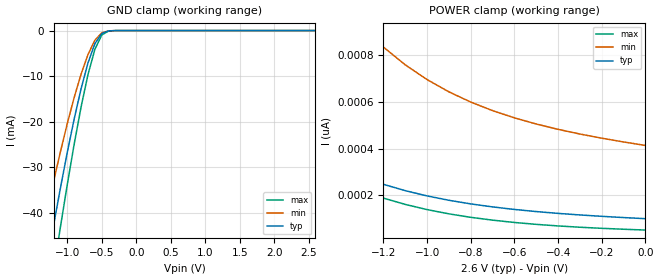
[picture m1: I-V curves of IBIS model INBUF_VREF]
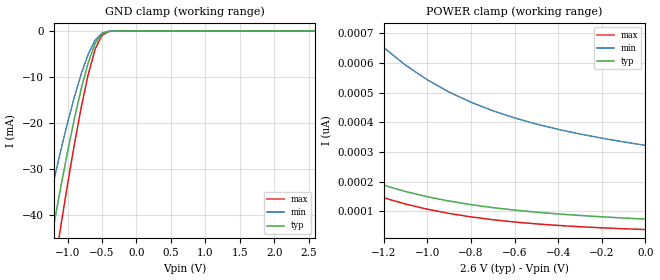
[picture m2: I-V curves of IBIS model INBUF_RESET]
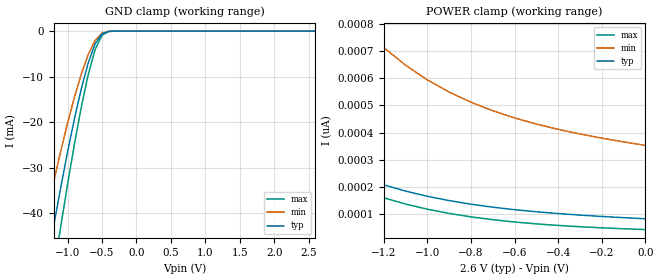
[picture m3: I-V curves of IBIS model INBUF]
| IBIS file sstvn859_tssop_3200.ibs created by s2ibis2 version 1.2
| North Carolina State University Electronics Research Laboratory  1995
[IBIS ver]   2.1
[File name]   sstvn859_tssop_3200.ibs
[File Rev]   1.0
[Date]   Thursday, November 6, 2003
[Source]   IDT
[Notes]   1. Temp typ=25C, min=0C, max=70C
   2. IDT's 2.0v C11.5 process
   3. Ramp rate based on 50 ohm load
READ THESE TERMS AND CONDITIONS CAREFULLY BEFORE USING THIS IBIS MODEL.  BY
USING THIS IBIS MODEL, YOU ARE ACCEPTING AND AGREEING TO THESE TERMS AND
CONDITIONS OF USE.
Integrated Device Technology, Inc. ("IDT") hereby grants the user of this
IBIS model ("User") a non-exclusive, nontransferable license to use this
IBIS model under the following terms: The User is granted this license only
to use the IBIS model for demonstration purposes only and is not granted
rights to sell, copy (except as needed to run the IBIS model), rent, lease
or sub-license (except for demonstration) the IBIS model in whole or in
part, or in modified form to anyone. The User may modify the IBIS model to
suit its specific applications, but  rights to derivative works and such
modifications shall belong to IDT.
THIS IBIS MODEL IS PROVIDED ON AN AS IS" BASIS AND IDT  MAKES ABSOLUTELY NO
WARRANTY WITH RESPECT TO THE INFORMATION CONTAINED HEREIN.  IDT DISCLAIMS
AND USER WAIVES ALL WARRANTIES, EXPRESS AND IMPLIED, INCLUDING WARRANTIES OF
MERCHANTABILITY AND FITNESS FOR A PARTICULAR PURPOSE.  THE ENTIRE RISK AS TO
QUALITY AND PERFORMANCE IS WITH THE USER  ACCORDINGLY, IN NO EVENT SHALL IDT
BE LIABLE FOR ANY DIRECT OR INDIRECT DAMAGES, WHETHER IN CONTRACT OR TORT,
INCLUDING ANY LOST PROFITS OR OTHER INCIDENTAL, CONSEQUENTIAL, EXEMPLARY, OR
PUNITIVE DAMAGES ARISING OUT OF THE USE OR APPLICATION OF THE  IBIS MODEL,
WHETHER OR NOT IDT HAD NOTICE OF SUCH DAMAGES.
IDT reserves the right to make changes without notice to any product herein
to improve reliability, function, or design. IDT does not convey any license
under patent rights or any other intellectual property rights, including
those of third parties. IDT is not obligated to provide maintenance or
support for the licensed IBIS model.
This model is for the 13-Bit to 26-Bit Registered Buffer With SSTL I/O
configuration
[Copyright]
Copyright 2002, Integrated Device Technology, Inc. All rights reserved.
|   Component IDT74SSTVN16859
[Component]   IDT74SSTVN16859
[Manufacturer]   Integrated Device Technology Inc.
[Package]
|Following package parameters are for TSSOP 64 lead package
| variable   typ   min   max
R_pkg   0.10500   68.00000m   0.14800
L_pkg   3.80000nH   2.05000nH   6.57000nH
C_pkg   0.22000pF   0.07183pF   0.42000pF
[Pin]  signal_name   model_name   R_pin   L_pin   C_pin
1   Q13A   OUTBUF
2   Q12A   OUTBUF
3   Q11A   OUTBUF
4   Q10A   OUTBUF
5   Q9A   OUTBUF
6   VDDQ   POWER
7   GND   GND
8   Q8A   OUTBUF
9   Q7A   OUTBUF
10   Q6A   OUTBUF
11   Q5A   OUTBUF
12   Q4A   OUTBUF
13   Q3A   OUTBUF
14   Q2A   OUTBUF
15   GND   GND
16   Q1A   OUTBUF
17   Q13B   OUTBUF
18   VDDQ   POWER
19   Q12B   OUTBUF
20   Q11B   OUTBUF
21   Q10B   OUTBUF
22   Q9B   OUTBUF
23   Q8B   OUTBUF
24   Q7B   OUTBUF
25   Q6B   OUTBUF
26   GND   GND
27   VDDQ   POWER
28   Q5B   OUTBUF
29   Q4B   OUTBUF
30   Q3B   OUTBUF
31   Q2B   OUTBUF
32   Q1B   OUTBUF
33   VDDQ   POWER
34   GND   GND
35   D1   INBUF
36   D2   INBUF
37   VDD   POWER
38   VDDQ   POWER
39   GND   GND
40   D3   INBUF
41   D4   INBUF
42   D5   INBUF
43   GND   GND
44   D6   INBUF
45   VREF   INBUF_VREF
46   VDD   POWER
47   VDDQ   POWER
48   CLK   INBUF_CLK
49   _CLK_   INBUF_CLK
50   GND   GND
51   _RESET_   INBUF_RESET
52   D7   INBUF
53   D8   INBUF
54   GND   GND
55   D9   INBUF
56   D10   INBUF
57   D11   INBUF
58   GND   GND
59   VDDQ   POWER
60   VDD   POWER
61   D12   INBUF
62   D13   INBUF
63   GND   INBUF
64   VDDQ   POWER
| in   in   dummy_model
[Diff Pin]  inv_pin  vdiff   tdelay_typ  tdelay_min  tdelay_max
48   49   0.36V   NA
[Pin Mapping]  pulldown_ref   pullup_ref   gnd_clamp_ref  power_clamp_ref
1   GND   VDDQ
2   GND   VDDQ
3   GND   VDDQ
4   GND   VDDQ
5   GND   VDDQ
6   NC   VDDQ
7   GND   NC
8   GND   VDDQ
9   GND   VDDQ
10   GND   VDDQ
11   GND   VDDQ
12   GND   VDDQ
13   GND   VDDQ
14   GND   VDDQ
15   GND   NC
16   GND   VDDQ
17   GND   VDDQ
18   NC   VDDQ
19   GND   VDDQ
20   GND   VDDQ
21   GND   VDDQ
22   GND   VDDQ
23   GND   VDDQ
24   GND   VDDQ
25   GND   VDDQ
26   GND   NC
27   NC   VDDQ
28   GND   VDDQ
29   GND   VDDQ
30   GND   VDDQ
31   GND   VDDQ
32   GND   VDDQ
33   NC   VDDQ
34   GND   NC
35   NC   NC   GND   VDDQ
36   NC   NC   GND   VDDQ
37   NC   VDD
38   NC   VDDQ
39   GND   NC
40   NC   NC   GND   VDDQ
41   NC   NC   GND   VDDQ
42   NC   NC   GND   VDDQ
43   GND   NC
44   NC   NC   GND   VDDQ
45   NC   NC   GND   VDDQ
46   NC   VDD
47   NC   VDDQ
48   NC   NC   GND   VDDQ
49   NC   NC   GND   VDDQ
50   GND   NC
51   NC   NC   GND   VDDQ
52   NC   NC   GND   VDDQ
53   NC   NC   GND   VDDQ
54   GND   NC
55   NC   NC   GND   VDDQ
56   NC   NC   GND   VDDQ
57   NC   NC   GND   VDDQ
58   GND   NC
59   NC   VDDQ
60   NC   VDD
61   NC   NC   GND   VDDQ
62   NC   NC   GND   VDDQ
63   NC   NC   GND   VDDQ
64   NC   VDDQ
| Models and submodels in the file (5): INBUF_VREF (Input), INBUF_RESET (Input), INBUF (Input), INBUF_CLK (Input), OUTBUF (Output)
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|   Model INBUF_VREF
[Model]   INBUF_VREF
Model_type   Input
Polarity   Non-Inverting
Vinl =  1.25000V
Vinh =  1.35000V
C_comp   2.50000pF   2.50000pF   2.50000pF
[Temperature Range]   25.00000   70.00000   0.000
[Voltage Range]   2.60000V   2.50000V   2.70000V
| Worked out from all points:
|   GND clamp passes 1 mA (typ) near -0.52 V on its own axis
[GND_clamp]
| voltage   I(typ)   I(min)   I(max)
-2.6V     -168.7mA   -138.9mA   -194.7mA
-1.4V     -60.05mA   -47.14mA   -72.86mA
-1.3V     -51.32mA   -40.05mA   -62.76mA
-1.2V     -42.8mA    -33.18mA   -52.81mA
-1.1V     -34.56mA   -26.6mA    -43.11mA
-900mV    -19.37mA   -14.66mA   -24.89mA
-800mV    -12.74mA   -9.544mA   -16.75mA
-700mV    -7.091mA   -5.252mA   -9.645mA
-600mV    -2.871mA   -2.118mA   -4.115mA
-500mV    -637.8uA   -495.3uA   -959.3uA
-300mV    -3.063uA   -4.006uA   -3.923uA
2.6V      98.9pA     428.4pA    47.06pA
[POWER_clamp]
| voltage   I(typ)   I(min)   I(max)
-2.6V     1.876nA    5.37nA     1.896nA
-2.2V     1.035nA    3.042nA    1.003nA
-2.1V     889.8pA    2.636nA    850.6pA
-2V       764.4pA    2.286nA    719.6pA
-1.9V     656.9pA    1.985nA    607.8pA
-1.7V     487pA      1.509nA    432.1pA
-1.5V     365.1pA    1.168nA    307.2pA
-1.3V     279.1pA    927.1pA    219.9pA
-1V       196.6pA    696.1pA    137.8pA
-800mV    162.4pA    599.6pA    104.7pA
-500mV    129.4pA    505.4pA    74.47pA
0V        98.9pA     413.4pA    50.09pA
|   Model INBUF_RESET
[Model]   INBUF_RESET
Model_type   Input
Polarity   Non-Inverting
Vinl =  0.70000V
Vinh =  1.70000V
C_comp   2.50000pF   2.50000pF   2.50000pF
[Temperature Range]   25.00000   70.00000   0.000
[Voltage Range]   2.60000V   2.50000V   2.70000V
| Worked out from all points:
|   GND clamp passes 1 mA (typ) near -0.52 V on its own axis
[GND_clamp]
| voltage   I(typ)   I(min)   I(max)
-2.6V     -167.2mA   -137.2mA   -193.3mA
-1.4V     -59.32mA   -46.36mA   -72.17mA
-1.3V     -50.66mA   -39.34mA   -62.13mA
-1.2V     -42.21mA   -32.55mA   -52.25mA
-1.1V     -34.04mA   -26.05mA   -42.6mA
-900mV    -18.98mA   -14.27mA   -24.51mA
-800mV    -12.43mA   -9.231mA   -16.44mA
-700mV    -6.859mA   -5.022mA   -9.408mA
-600mV    -2.718mA   -1.972mA   -3.951mA
-500mV    -567.1uA   -431.8uA   -874.7uA
-300mV    -2.396uA   -3.132uA   -3.069uA
2.6V      74.28pA    334.2pA    36.7pA
[POWER_clamp]
| voltage   I(typ)   I(min)   I(max)
-2.6V     1.459nA    4.19nA     1.48nA
-2.2V     802.9pA    2.373nA    783.1pA
-2.1V     689.4pA    2.056nA    663.8pA
-2V       591.6pA    1.783nA    561.6pA
-1.9V     507.7pA    1.549nA    474.3pA
-1.7V     375.3pA    1.178nA    337.2pA
-1.5V     280.4pA    911.3pA    239.7pA
-1.3V     213.5pA    723.3pA    171.6pA
-1V       149.5pA    543.1pA    107.5pA
-800mV    122.9pA    467.8pA    81.69pA
-500mV    97.55pA    394.3pA    58.09pA
0V        74.28pA    322.6pA    39.06pA
|   Model INBUF
[Model]   INBUF
Model_type   Input
Polarity   Non-Inverting
Vinl =  0.94000V
Vinh =  1.66000V
C_comp   2.50000pF   2.50000pF   2.50000pF
[Temperature Range]   25.00000   70.00000   0.000
[Voltage Range]   2.60000V   2.50000V   2.70000V
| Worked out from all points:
|   GND clamp passes 1 mA (typ) near -0.52 V on its own axis
[GND_clamp]
| voltage   I(typ)   I(min)   I(max)
-2.6V     -168.1mA   -138.2mA   -194.1mA
-1.4V     -59.73mA   -46.79mA   -72.56mA
-1.3V     -51.03mA   -39.73mA   -62.48mA
-1.2V     -42.53mA   -32.89mA   -52.56mA
-1.1V     -34.32mA   -26.35mA   -42.88mA
-900mV    -19.19mA   -14.47mA   -24.71mA
-800mV    -12.59mA   -9.39mA    -16.6mA
-700mV    -6.975mA   -5.134mA   -9.529mA
-600mV    -2.79mA    -2.039mA   -4.03mA
-500mV    -596.8uA   -457.6uA   -911.7uA
-300mV    -2.619uA   -3.425uA   -3.355uA
2.6V      82.49pA    365.6pA    40.15pA
[POWER_clamp]
| voltage   I(typ)   I(min)   I(max)
-2.6V     1.598nA    4.583nA    1.618nA
-2.2V     880.4pA    2.596nA    856.5pA
-2.1V     756.2pA    2.249nA    726.1pA
-2V       649.2pA    1.951nA    614.3pA
-1.9V     557.4pA    1.694nA    518.8pA
-1.7V     412.5pA    1.288nA    368.8pA
-1.5V     308.6pA    996.8pA    262.2pA
-1.3V     235.3pA    791.2pA    187.7pA
-1V       165.2pA    594.1pA    117.6pA
-800mV    136.1pA    511.7pA    89.36pA
-500mV    108.2pA    431.3pA    63.55pA
0V        82.49pA    352.8pA    42.73pA
